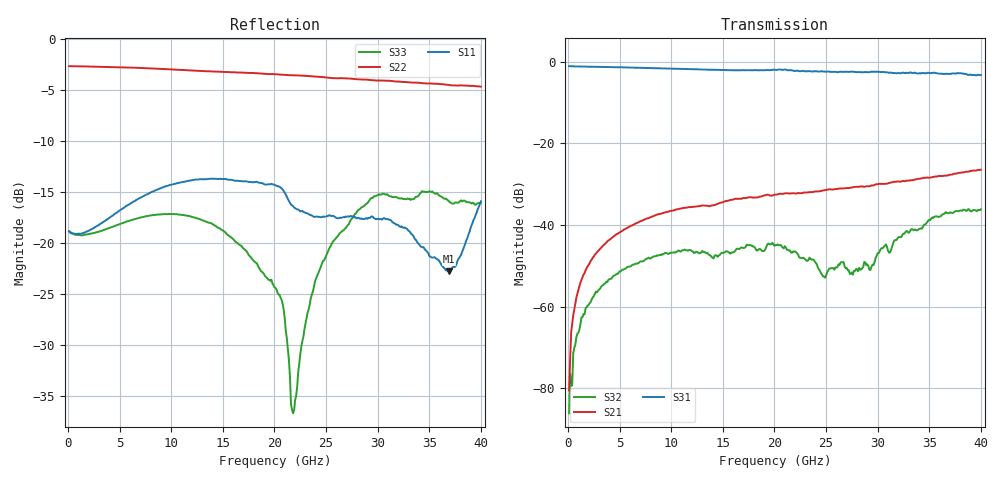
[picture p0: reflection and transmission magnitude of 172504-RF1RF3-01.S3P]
!  3-Port S-parameters saved by WinCal
! VAR MeasName=S-Parameters (CALIBRATED_DATA) read from VNA (N5245A)
! VAR MeasDate=2017-3-15 11:07:41
! VAR NAME=172504-RF1RF3-01
! VAR FILENAME=172504-RF1RF3-01.S3P
! VAR DATE=2017-3-15 11:07:41
! VAR PHYS_PORTS=1,2,3
# Hz S DB R 50
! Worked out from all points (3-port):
!   400 points, 100 MHz to 40 GHz, reference 50 ohm
!   strongest paths, dB at 100 MHz, 10.1 GHz, 20.1 GHz, 30.1 GHz, 40 GHz:
!     S31: -1.1, -1.7, -2.0, -2.5, -3.3
!     S21: -80.5, -36.5, -32.6, -30.0, -26.5
!     S32: -86.1, -46.8, -44.9, -46.9, -36.1
!   lowest |S11| = -22.8 dB at 36.9 GHz (marker M1), VSWR 1.16, Z = 46.7 + j6.24 ohm
!   |S11| at or under -10 dB: start of sweep to end of sweep
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1e8  -18.84 -2.7  -79.16 135.1  -1.10 -0.8
     -80.49 65.2  -2.65 179.8  -85.43 147.3
     -1.10 -0.8  -86.11 -167.8  -18.86 -2.4
3e8  -19.00 -6.5  -66.09 100.0  -1.13 -2.1
     -66.17 97.6  -2.66 179.3  -75.66 96.4
     -1.13 -2.1  -79.44 123.9  -19.04 -5.8
1e9  -19.08 -18.3  -55.72 91.0  -1.17 -6.5
     -55.77 90.3  -2.67 177.8  -66.09 97.9
     -1.18 -6.5  -66.37 101.4  -19.21 -16.1
3.8e9  -17.67 -56.6  -44.05 71.9  -1.32 -23.4
       -44.02 71.8  -2.73 172.0  -53.56 66.4
       -1.32 -23.4  -53.96 66.3  -18.61 -52.1
2.01e10  -14.34 -150.1  -32.30 -5.4  -2.00 -117.0
         -32.57 -4.0  -3.45 137.9  -45.15 -50.6
         -2.02 -116.8  -44.91 -54.4  -24.42 -146.0
2.18e10  -16.38 -156.1  -32.26 -15.0  -2.37 -129.1
         -32.22 -13.0  -3.55 134.1  -46.11 -69.3
         -2.21 -128.8  -46.46 -70.4  -36.70 -118.6
2.57e10  -17.33 -147.1  -31.32 -29.3  -2.55 -150.3
         -31.26 -27.5  -3.83 124.4  -50.11 -65.7
         -2.47 -150.2  -50.58 -65.5  -19.81 -60.4
2.76e10  -17.39 -147.3  -30.80 -37.4  -2.67 -161.5
         -30.75 -35.4  -3.90 119.5  -53.21 -60.7
         -2.47 -161.7  -52.16 -55.2  -17.43 -66.0
3.69e10  -22.78 113.8  -27.68 -87.7  -3.08 139.5
         -27.74 -84.8  -4.49 92.7  -37.84 -102.1
         -3.01 140.0  -37.10 -106.0  -15.91 -95.3
4e10  -15.91 40.3  -26.32 -108.2  -3.27 118.4
      -26.45 -107.6  -4.67 82.6  -36.50 -130.8
      -3.26 118.0  -36.14 -137.5  -16.03 -85.2
